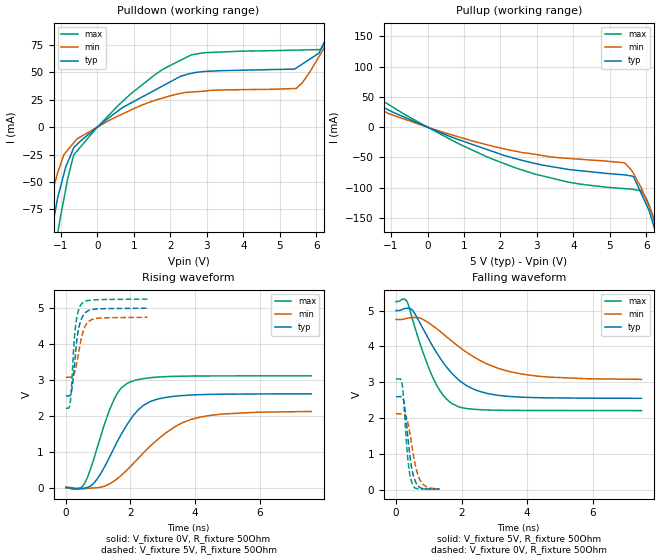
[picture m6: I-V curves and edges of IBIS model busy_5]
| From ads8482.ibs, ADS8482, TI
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|   busy_5 Model
[Model]   busy_5
Model_type   Output
Polarity   Non-Inverting
Vmeas = 2.5
Vref = 2.5
Cref = 5pF
Rref = 50
|   typ   min   max
|   (nom PVT)   (Fast PVT)   (slow PVT)
|C_comp from frequency method(F=1MHz)
|Average
|C_comp   3.575e-11   1.863e-11   6.834e-11
|ON state : BUFFER OUTPUT TURNED HIGH
|C_comp   3.575e-11   1.863e-11   6.834e-11
|OFF state: BUFFER OUTPUT TURNED LOW
|C_comp   4.500e-12   3.828e-12   5.438e-12
|C_comp from L-C Tank method(L=1nH)
|Resonant Frequency(Hz)   3.57e9   4.04e9   3.22e9
C_comp   1.989e-12   1.553e-12  2.445e-12
| Where nom  PVT is Nominal Process,  5V,  30C
|   Fast PVT is Strong Process,   5.25V,  -40C
|   Slow PVT is Weak Process,   4.75V,  90C
[Voltage Range]   5   4.75   5.25
|Ambient Temperature   25   85   -40
|Junction Temperature
[Temperature Range]   30   90   -40
[Pullup Reference]   5   4.75   5.25
[Pulldown Reference]   0   0   0
[Power Clamp Reference]   5   4.75   5.25
[GND Clamp Reference]   0   0   0
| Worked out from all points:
|   slope of the pulldown table from 0 to 0.75 V, typ, clamps not added: 39.6 ohm
|   slope of the pullup table from 0 to 0.75 V, typ, clamps not added: 40.6 ohm
|   falling waveform, V_fixture 5V, R_fixture 50Ohm: 20-80 % time 1.13ns typ, 1.69ns min, 766ps max; typ from 5 V to 2.55 V
|   rising waveform, V_fixture 0V, R_fixture 50Ohm: 20-80 % time 1ns typ, 1.56ns min, 710ps max; typ from 0 V to 2.61 V
|   rising waveform, V_fixture 5V, R_fixture 50Ohm: 20-80 % time 188ps typ, 233ps min, 146ps max; typ from 2.55 V to 4.99 V
|   falling waveform, V_fixture 0V, R_fixture 50Ohm: 20-80 % time 197ps typ, 259ps min, 152ps max; typ from 2.6 V to 0.019 V
[Pulldown]
|   Voltage   I(typ)   I(min)   I(max)
-5V       -952.4mA   -696.2mA   -1.294A
-1.838V   -221.8mA   -145.6mA   -312.1mA
-1.302V   -104mA     -67.97mA   -149.2mA
-1.085V   -64.27mA   -41.46mA   -96.91mA
-916.7mV  -42.87mA   -25.18mA   -65.67mA
-640.5mV  -18.51mA   -14.02mA   -25.06mA
924mV     22.09mA    15.66mA    30.63mA
2.578V    49.16mA    32.08mA    66.05mA
5.453V    54.03mA    35.31mA    70.36mA
6.132V    71.62mA    67.65mA    71.31mA
6.564V    102.1mA    91.92mA    103.8mA
10V       254mA      213.5mA    302mA
[Pullup]
|   Voltage   I(typ)   I(min)   I(max)
-5V       174.6mA    156.3mA    199.3mA
-3.791V   151.1mA    133mA      175.5mA
-3.019V   128mA      110.5mA    150.1mA
-1.554V   51.02mA    43.74mA    58.45mA
-190mV    4.947mA    3.863mA    6.353mA
2.94V     -59.91mA   -44.87mA   -77.47mA
5.396V    -78.79mA   -58.81mA   -101.5mA
5.645V    -81.64mA   -76.63mA   -103mA
5.864V    -110.5mA   -101.5mA   -105.4mA
6.179V    -159.1mA   -146.5mA   -147.6mA
6.3V      -183.3mA   -163.8mA   -177.6mA
10V       -1.043A    -807.5mA   -1.328A
[Ramp]
R_load = 50
|   typ   min   max
dV/dt_r   1.56531/1.00139e-09   1.27416/1.57095e-09   1.86537/7.09787e-10
dV/dt_f   1.47069/1.13016e-09   1.00576/1.70638e-09   1.82562/7.653e-10
[Falling Waveform]
V_fixture = 5V
V_fixture_min = 4.75V
V_fixture_max = 5.25V
R_fixture = 50Ohm
|   Time   V(typ)   V(min)   V(max)
0s        5V         4.75V      5.25V
334ps     5.063V     4.784V     5.255V
511ps     4.999V     4.804V     4.732V
819ps     4.503V     4.754V     3.843V
1.177ns   3.918V     4.538V     3.03V
1.528ns   3.441V     4.279V     2.543V
1.904ns   3.071V     4.002V     2.317V
2.737ns   2.697V     3.528V     2.227V
3.853ns   2.582V     3.225V     2.212V
7.492ns   2.551V     3.08V      2.208V
[Rising Waveform]
V_fixture = 0V
V_fixture_min = 0V
V_fixture_max = 0V
R_fixture = 50Ohm
|   Time   V(typ)   V(min)   V(max)
0s        1.46nV     1.714nV    1.291nV
568ps     -17.21mV   -33.83mV   92.6mV
953ps     215.9mV    -6.345mV   1.049V
1.493ns   1.096V     179.5mV    2.447V
1.7ns     1.453V     325.7mV    2.751V
1.962ns   1.841V     548.7mV    2.927V
2.611ns   2.391V     1.152V     3.056V
3.875ns   2.575V     1.895V     3.103V
4.882ns   2.599V     2.048V     3.107V
7.601ns   2.608V     2.117V     3.109V
[Rising Waveform]
V_fixture = 5V
V_fixture_min = 4.75V
V_fixture_max = 5.25V
R_fixture = 50Ohm
|   Time   V(typ)   V(min)   V(max)
0s        2.548V     3.071V     2.207V
101ps     2.549V     3.071V     2.221V
138ps     2.573V     3.071V     2.367V
206ps     2.84V      3.096V     3.262V
283ps     3.548V     3.248V     4.343V
363ps     4.248V     3.578V     4.829V
467ps     4.649V     4.095V     5.089V
609ps     4.868V     4.509V     5.189V
818ps     4.956V     4.679V     5.219V
2.528ns   4.992V     4.739V     5.245V
[Falling Waveform]
V_fixture = 0V
V_fixture_min = 0V
V_fixture_max = 0V
R_fixture = 50Ohm
|   Time   V(typ)   V(min)   V(max)
0s        2.595V     2.117V     3.089V
134ps     2.597V     2.117V     3.092V
190ps     2.574V     2.117V     2.938V
256ps     2.372V     2.1V       2.224V
356ps     1.537V     1.898V     903.5mV
419ps     988.4mV    1.602V     451mV
498ps     516.1mV    1.155V     161.4mV
622ps     174mV      560.9mV    34.14mV
758ps     48.5mV     232mV      22.06mV
1.326ns   18.66mV    19.59mV    15.61mV
